FUNCTION_BLOCK FB 29
TITLE =
//
AUTHOR : NUMERIK
FAMILY : _800D
NAME : Diag
VERSION : 1.0
CODE_VERSION1


VAR_INPUT
  Func : INT ;	//Function number
//0 = No Function, 1 = Signalrecorder, 2 = Datatrigger
  Signal_1 : BOOL ;
  Signal_2 : BOOL ;
  Signal_3 : BOOL ;
  Signal_4 : BOOL ;
  Signal_5 : BOOL ;
  Signal_6 : BOOL ;
  Signal_7 : BOOL ;
  Signal_8 : BOOL ;
  NewCycle : BOOL ;
  Var1 : BYTE ;
  Var2 : INT ;
  Var3 : INT ;
  BufDB : INT ;
  ClearBuf : BOOL ;
  DataAdr : POINTER ;	//Area pointer to testing word
  TestVal : WORD ;	//Value for triggering
  AndMask : WORD ;	//AND- Mask to the testing word
END_VAR
VAR_OUTPUT
  TestIsTrue : BOOL ;
END_VAR
VAR_IN_OUT
  BufAddr : INT ;
END_VAR
VAR
  Cycle : INT ;
  edgePN : ARRAY  [0 .. 15 ] OF BOOL ;
  BufPtr : DWORD ;
  reset_edge : BOOL ;
END_VAR
VAR_TEMP
  dbtest : WORD ;
  value : WORD ;
  return : INT ;
  dest : ANY ;
END_VAR
BEGIN
NETWORK
TITLE =

      L     #Func; //Function
      SPL   z009;
      SPA   z009;
      SPA   z001;
      SPA   z002;
z009: BEA   ;
NETWORK
TITLE = Function 1

z001: AUF   DB [#BufDB]; //DB RingBuffer
      U     #ClearBuf; //Clear the buffer
      FP    #reset_edge;
      SPBN  goon;
      L     B#16#0; //clear value
      T     #value;
      T     #Cycle;
      LAR1  P##dest;
//make variable ANY of whole BufDB
      L     W#16#1004; //Type = WORD (04)
      T     LW [AR1,P#0.0];
      L     DBLG; //length of Buffer-DB
      SRW   1; //in WORDs
      T     LW [AR1,P#2.0];
      L     #BufDB; //DB-Number
      T     LW [AR1,P#4.0];
      L     P#DBX 0.0; //Offset in DB = 0
      T     LD [AR1,P#6.0];
      CALL  SFC 21 (//clear the Buffer
           BVAL                     := #value,
           RET_VAL                  := #return,
           BLK                      := #dest);

      SPA   res;
goon: U     #NewCycle; //if new cycle
      SPBN  m400;
      L     #Cycle; //Increment of cycle counter
      +     1;
      T     #Cycle;
m400: LAR1  P##Signal_1; //Test any edge of signals
      LAR2  P##edgePN;
      L     DIB [AR1,P#0.0]; //Signals
      L     DIB [AR2,P#0.0]; //edge buffer
      XOW   ;
      SPZ   end1; //no edge
      TAK   ;
      T     DIB [AR2,P#0.0]; //to edge buffer
      LAR2  #BufPtr;
      T     DBB [AR2,P#2.0]; //Signals to RingBuffer
      L     #Cycle;
      T     DBW [AR2,P#0.0]; //Delta cycle count to RingBuffer
      L     #Var1;
      T     DBB [AR2,P#3.0]; //Var1 to RingBuffer
      L     #Var2;
      T     DBW [AR2,P#4.0]; //Var2 to RingBuffer
      L     #Var3;
      T     DBW [AR2,P#6.0]; //Var3 to RingBuffer
      L     B#16#0; //Clear cycle counter
      T     #Cycle;
      +AR2  P#8.0; //next offset in Buffer
      TAR2  ;
      T     #BufPtr;
      SRD   3;
      T     #BufAddr;
      L     DBLG; //max. length of Buffer
      ==I   ;
      SPBN  end1;
res:  L     B#16#0; //Buffer-Pointer to Zero
      T     #BufPtr;
      T     #BufAddr;
end1: BEA   ;

NETWORK
TITLE = Function 2

z002: LAR1  P##DataAdr; //catch Pointer
      L     DIW [AR1,P#0.0];
      T     #dbtest;
      L     DID [AR1,P#2.0];
      LAR1  ;
      AUF   DB [#dbtest]; //DB of testing word
      L     W [AR1,P#0.0]; //load testing word
      L     #AndMask;
      UW    ; //mask it
      L     #TestVal;
      ==I   ; //compare it after masking
      =     #TestIsTrue; //error in TestIsTrue

END_FUNCTION_BLOCK


DATA_BLOCK DB 80
TITLE =
//Instanz-DB FB 29
VERSION : 1.0

 FB 29
BEGIN
END_DATA_BLOCK

//******************************

//must be a DB from the User Area

DATA_BLOCK DB 81
TITLE =
//Ring buffer-DB for FB 29
VERSION : 1.0


  STRUCT
   Feld : ARRAY  [0 .. 249 ] OF STRUCT 	//can be any size of this struct
    Cycle : INT ;	//Delta cycle to last storage in buffer
    Signal_1 : BOOL ;	//Signal names same as FB 29
    Signal_2 : BOOL ;
    Signal_3 : BOOL ;
    Signal_4 : BOOL ;
    Signal_5 : BOOL ;
    Signal_6 : BOOL ;
    Signal_7 : BOOL ;
    Signal_8 : BOOL ;
    Var1 : BYTE ;
    Var2 : WORD ;
    Var3 : WORD ;
   END_STRUCT ;
  END_STRUCT ;
BEGIN
END_DATA_BLOCK

//Example for use


FUNCTION FC 99: VOID
TITLE =
VERSION : 0.0

BEGIN
NETWORK
TITLE =   NETWORK

      CALL FB    29 , DB    80 (
           Func                     := 1,
           Signal_1                 := M    100.0,
           Signal_2                 := M    100.1,
           Signal_3                 := M    100.2,
           Signal_4                 := M    100.3,
           Signal_5                 := M    100.4,
           Signal_6                 := M    100.5,
           Signal_7                 := M    100.6,
           Signal_8                 := M    100.7,
           NewCycle                 := TRUE,
           Var1                     := MB   100,
           BufDB                    := 81,
           ClearBuf                 := M     50.0);

END_FUNCTION

